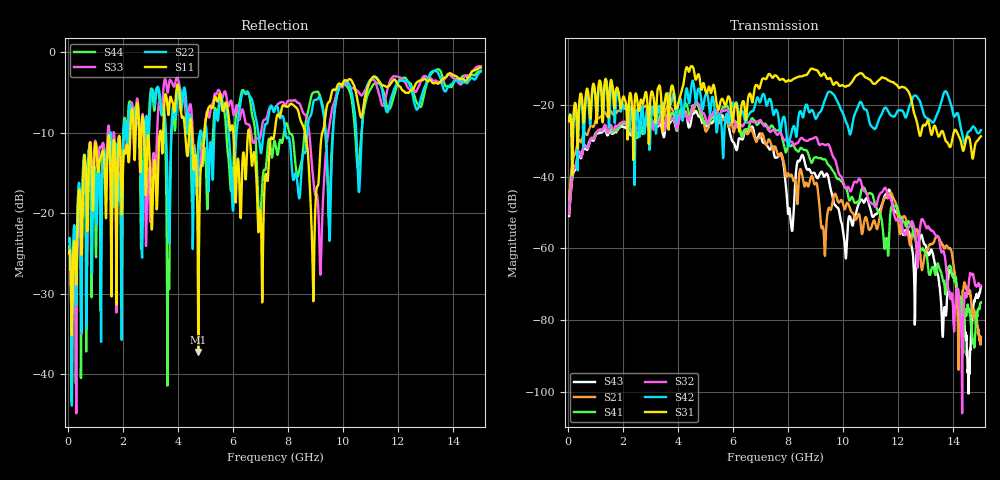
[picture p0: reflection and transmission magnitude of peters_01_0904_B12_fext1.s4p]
# MHZ S RI R 50.00
! FREQ  S11  S12  S13  S14
!  S21  S22  S23  S24
!  S31  S32  S33  S34
!  S41  S42  S43  S44
!  REAL  IMAG  REAL  IMAG  REAL  IMAG  REAL  IMAG
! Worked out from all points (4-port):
!   1496 points, 50 MHz to 15 GHz, reference 50 ohm
!   strongest paths, dB at 50 MHz, 3.79 GHz, 7.53 GHz, 11.27 GHz, 15 GHz:
!     S31: -24.5, -14.5, -11.7, -13.2, -28.7
!     S42: -24.3, -18.5, -21.7, -24.6, -27.0
!     S32: -50.4, -23.7, -27.6, -46.1, -70.5
!     S41: -50.2, -22.2, -26.9, -49.8, -75.0
!     S21: -46.7, -21.2, -31.6, -53.7, -84.9
!     S43: -51.0, -24.1, -34.7, -49.6, -70.8
!   lowest |S11| = -37.2 dB at 4.74 GHz (marker M1), VSWR 1.03, Z = 50.1 + j1.38 ohm
!   |S11| at or under -10 dB: start of sweep to 2.272 GHz; 6.6 GHz to 7.511 GHz (911 MHz wide, 12.9 % of centre); 8.612 GHz to 9.242 GHz (629.4 MHz wide, 7.05 % of centre)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
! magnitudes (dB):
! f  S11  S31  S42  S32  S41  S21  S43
! 50 MHz  -25.0  -24.5  -24.3  -50.4  -50.2  -46.7  -51.0
! 3.25 GHz  -18.5  -16.5  -22.7  -25.2  -24.4  -21.7  -25.8
! 3.65 GHz  -7.8  -24.2  -16.8  -23.0  -23.4  -20.4  -24.2
! 3.99 GHz  -4.0  -20.4  -20.7  -26.1  -26.4  -25.2  -25.8
! 4.74 GHz  -37.2  -11.4  -15.4  -19.7  -20.1  -20.1  -23.0
! 11.75 GHz  -3.8  -13.5  -23.0  -46.8  -48.4  -44.6  -45.7
! 15 GHz  -1.9  -28.7  -27.0  -70.5  -75.0  -84.9  -70.8
